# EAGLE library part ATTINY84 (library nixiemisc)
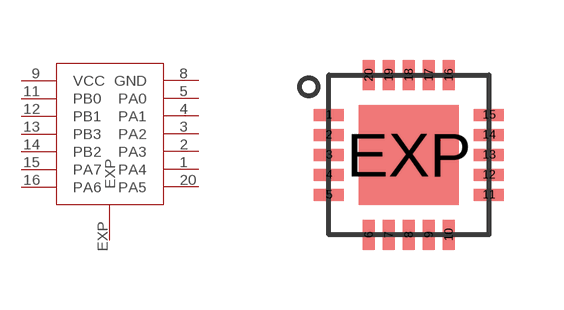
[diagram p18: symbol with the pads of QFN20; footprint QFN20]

Designator prefix M

## ATTINY84  [QFN20]
1  PA4  pas
2  PA3  pas
3  PA2  pas
4  PA1  pas
5  PA0  pas
8  GND  pwr
9  VCC  pwr
11  PB0  pas
12  PB1  pas
13  PB3  pas
14  PB2  pas
15  PA7  pas
16  PA6  pas
20  PA5  pas
EXP  EXP  pwr

## Footprint QFN20 (pad centres in mm)
smd 0.75 x 0.3: 1 -2,1; 2 -2,0.5; 3 -2,0; 4 -2,-0.5; 5 -2,-1; 11 2,-1; 12 2,-0.5; 13 2,0; 14 2,0.5; 15 2,1
smd 0.3 x 0.75: 6 -1,-2; 7 -0.5,-2; 8 0,-2; 9 0.5,-2; 10 1,-2; 16 1,2; 17 0.5,2; 18 0,2; 19 -0.5,2; 20 -1,2
smd 2.5 x 2.5: EXP 0,0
